| IBIS file stm32h562_563_573_ufbga201.ibs
[IBIS ver] 4.2
[File name] stm32h562_563_573_ufbga201.ibs
[File Rev] 1.1
[Date] 07-05-2024
[Source] Data Created at STMicroelectronics
[Notes]  File originated from ELDO simulations.
[Disclaimer]  This information is for modeling purpose only and is
   not guaranteed. The information is subject to change without
   notice.
[Copyright] Copyright 2024 STMicroelectronics Inc.
|   Component stm32h562_563_573_ufbga201
[Component] stm32h562_563_573_ufbga201
[Manufacturer] STMicroelectronics
[Package]
| variable   typ   min   max
R_pkg  0  NA  NA
L_pkg  0  NA  NA
C_pkg  0  NA  NA
[Pin]   signal_name   model_name
A1  PE3  io8_ft_i3c_spi
A2  PE2  io8_ft_i3c_spi
A3  PE1  io8_ft_i3c_spi
A4  PE0  io8_ft_i3c_spi
A5  PB8  io8_ft_i3c_spi
A6  PB5  io8_ft_i3c_spi
A7  PG14  io8_ft_i3c_spi
A8  PG13  io8_ft_i3c_spi
A9  PB4  io8_ft_i3c_spi
A10  PB3  io8_ft_i3c_spi
A11  PD7  io8_ft_i3c_spi
A12  PC12  io8_ft_i3c_spi
A13  PA15  io8_ft_i3c_spi
A14  PA14  io8_ft_i3c_spi
A15  PA13  io8_ft_i3c_spi
B1  PE4  io8_ft_i3c_spi
B2  PE5  io8_ft_i3c_spi
B3  PE6  io8_ft_i3c_spi
B4  PB9  io8_ft_i3c_spi
B5  PB7  io8_ft_i3c_spi
B6  PB6  io8_ft_i3c_spi
B7  PG15  io8_ft_i3c_spi
B8  PG12  io8_ft_i3c_spi
B9  PG11  io8_ft_i3c_spi
B10  PG10  io8_ft_i3c_spi
B11  PD6  io8_ft_i3c_spi
B12  PD0  io8_ft_i3c_spi
B13  PC11  io8_ft_i3c_spi
B14  PC10  io8_ft_i3c_spi
B15  PA12  io8usb_ft_i3c_spi_phy
C1  VBAT  power
C2  PI7  io8_ft_i3c_spi
C3  PI6  io8_ft_i3c_spi
C4  PI5  io8_ft_i3c_spi
C5  VDD  power
C6  VCAP  nc
C7  VDD  power
C8  VDDIO2  power
C9  VDD  power
C10  PG9  io8_ft_i3c_spi
C11  PD5  io8_ft_i3c_spi
C12  PD1  io8_ft_i3c_spi
C13  PI3  io8_ft_i3c_spi
C14  PI2  io8_ft_i3c_spi
C15  PA11  io8usb_ft_i3c_spi_phy
D1  PC13  io8_ft_i3c_spi
D2  PI8  io8_ft_i3c_spi
D3  PI9  io8_ft_i3c_spi
D4  PI4  io8_ft_i3c_spi
D5  VSS  gnd
D6  BOOT0  vpphv
D7  VSS  gnd
D8  VSS  gnd
D9  VSS  gnd
D10  PD4  io8_ft_i3c_spi
D11  PD3  io8_ft_i3c_spi
D12  PD2  io8_ft_i3c_spi
D13  PH15  io8_ft_i3c_spi
D14  PI1  io8_ft_i3c_spi
D15  PA10  io8_ft_i3c_spi
E1  PC14-OSC32_IN  io8_ft_i3c_spi
E2  PF0  io8_ft_i3c_spi
E3  PI10  io8_ft_i3c_spi
E4  PI11  io8_ft_i3c_spi
E12  PH13  io8_ft_i3c_spi
E13  PH14  io8_ft_i3c_spi
E14  PI0  io8_ft_i3c_spi
E15  PA9  io8_ft_i3c_spi
F1  PC15-OSC32_OUT  io8_ft_i3c_spi
F2  VSS  gnd
F3  VDD  power
F4  PH2  io8_ft_i3c_spi
F6  VSS  gnd
F7  VSS  gnd
F8  VSS  gnd
F9  VSS  gnd
F10  VSS  gnd
F12  VSS  gnd
F13  VDD  power
F14  PC9  io8_ft_i3c_spi
F15  PA8  io8_ft_i3c_spi
G1  PH0-OSC_IN  io8_ft_i3c_spi
G2  VSS  gnd
G3  VDD  power
G4  PH3  io8_ft_i3c_spi
G6  VSS  gnd
G7  VSS  gnd
G8  VSS  gnd
G9  VSS  gnd
G10  VSS  gnd
G12  VSS  gnd
G13  VDD  power
G14  PC8  io8_ft_i3c_spi
G15  PC7  io8_ft_i3c_spi
H1  PH1-OSC_OUT  io8_ft_i3c_spi
H2  PF2  io8_ft_i3c_spi
H3  PF1  io8_ft_i3c_spi
H4  PH4  io8_ft_i3c_spi
H6  VSS  gnd
H7  VSS  gnd
H8  VSS  gnd
H9  VSS  gnd
H10  VSS  gnd
H12  VSS  gnd
H13  VDDUSB  power
H14  PG8  io8_ft_i3c_spi
H15  PC6  io8_ft_i3c_spi
J1  NRST  ioreset_ft_v33
J2  PF3  io8_ft_i3c_spi
J3  PF4  io8_ft_i3c_spi
J4  PH5  io8_ft_i3c_spi
J6  VSS  gnd
J7  VSS  gnd
J8  VSS  gnd
J9  VSS  gnd
J10  VSS  gnd
J12  VDD  power
J13  VDD  power
J14  PG7  io8_ft_i3c_spi
J15  PG6  io8_ft_i3c_spi
K1  PF7  io8_ft_i3c_spi
K2  PF6  io8_ft_i3c_spi
K3  PF5  io8_ft_i3c_spi
K4  VDD  power
K6  VSS  gnd
K7  VSS  gnd
K8  VSS  gnd
K9  VSS  gnd
K10  VSS  gnd
K12  PH12  io8_ft_i3c_spi
K13  PG5  io8_ft_i3c_spi
K14  PG4  io8_ft_i3c_spi
K15  PG3  io8_ft_i3c_spi
L1  PF10  io8_ft_i3c_spi
L2  PF9  io8_ft_i3c_spi
L3  PF8  io8_ft_i3c_spi
L4  VSS  gnd
L12  PH11  io8_ft_i3c_spi
L13  PH10  io8_ft_i3c_spi
L14  PD15  io8_ft_i3c_spi
L15  PG2  io8_ft_i3c_spi
M1  VSSA  nc
M2  PC0  io8_ft_spi
M3  PC1  io8_ft_spi
M4  PC2  io8_ft_spi
M5  PC3  io8_ft_spi
M6  PB2  io8_ft_i3c_spi
M7  PG1  io8_ft_i3c_spi
M8  VSS  gnd
M9  VSS  gnd
M10  VCAP  nc
M11  PH6  io8_ft_i3c_spi
M12  PH8  io8_ft_i3c_spi
M13  PH9  io8_ft_i3c_spi
M14  PD14  io8_ft_i3c_spi
M15  PD13  io8_ft_i3c_spi
N1  VREFM  nc
N2  PA1  io8_ft_spi_tamp
N3  PA0  io8_ft_spi
N4  PA4  io8_ft_spi
N5  PC4  io8_ft_spi
N6  PF13  io8_ft_spi
N7  PG0  io8_ft_i3c_spi
N8  VDD  power
N9  VDD  power
N10  VDD  power
N11  PE13  io8_ft_i3c_spi
N12  PH7  io8_ft_i3c_spi
N13  PD12  io8_ft_i3c_spi
N14  PD11  io8_ft_i3c_spi
N15  PD10  io8_ft_i3c_spi
P1  VREFP  nc
P2  PA2  io8_ft_spi
P3  PA6  io8_ft_spi
P4  PA5  io8_ft_spi
P5  PC5  io8_ft_spi
P6  PF12  io8_ft_spi
P7  PF15  io8_ft_i3c_spi
P8  PE8  io8_ft_i3c_spi
P9  PE9  io8_ft_i3c_spi
P10  PE11  io8_ft_i3c_spi
P11  PE14  io8_ft_i3c_spi
P12  PB12  io8_ft_i3c_spi
|P13  PB13  io8usb_ft_pd
P13  PB13  nc
P14  PD9  io8_ft_i3c_spi
P15  PD8  io8_ft_i3c_spi
R1  VDDA  nc
R2  PA3  io8_ft_spi
R3  PA7  io8_ft_spi
R4  PB1  io8_ft_spi
R5  PB0  io8_ft_spi
R6  PF11  io8_ft_spi
R7  PF14  io8_ft_spi
R8  PE7  io8_ft_i3c_spi
R9  PE10  io8_ft_i3c_spi
R10  PE12  io8_ft_i3c_spi
R11  PE15  io8_ft_i3c_spi
R12  PB10  io8_ft_i3c_spi
R13  PB11  io8_ft_i3c_spi
|R14  PB14  io8usb_ft_pd
R14  PB14  nc
R15  PB15  io8_ft_spi
[Package Model]   484-ufbga-10x10-201-ldo-221014
[Pin Mapping]   pulldown_ref   pullup_ref   | Comment
A1  gndio  vddiom
A2  gndio  vddiom
A3  gndio  vddiom  | Depending on IO usage
| A3  gndio  vddmmc  | Depending on IO usage
A4  gndio  vddiom  | Depending on IO usage
| A4  gndio  vddmmc  | Depending on IO usage
A5  gndio  vddiom  | Depending on IO usage
| A5  gndio  vddmmc  | Depending on IO usage
A6  gndio  vddiom  | Depending on IO usage
| A6  gndio  vddmmc  | Depending on IO usage
A7  gndio  vddiom  | Depending on IO usage
| A7  gndio  vddmmc  | Depending on IO usage
A8  gndio  vddiom  | Depending on IO usage
| A8  gndio  vddmmc  | Depending on IO usage
A9  gndio  vddiom  | Depending on IO usage
| A9  gndio  vddmmc  | Depending on IO usage
A10  gndio  vddiom  | Depending on IO usage
| A10  gndio  vddmmc  | Depending on IO usage
A11  gndio  vddiom  | Depending on IO usage
| A11  gndio  vddmmc  | Depending on IO usage
A12  gndio  vddiom
A13  gndio  vddiom
A14  gndio  vddiom
A15  gndio  vddiom  | Depending on IO usage
| A15  gndio  vddusb  | Depending on IO usage
B1  gndio  vddiom
B2  gndio  vddiom
B3  gndio  vddiom
B4  gndio  vddiom  | Depending on IO usage
| B4  gndio  vddmmc  | Depending on IO usage
B5  gndio  vddiom  | Depending on IO usage
| B5  gndio  vddmmc  | Depending on IO usage
B6  gndio  vddiom  | Depending on IO usage
| B6  gndio  vddmmc  | Depending on IO usage
B7  gndio  vddiom  | Depending on IO usage
| B7  gndio  vddmmc  | Depending on IO usage
B8  gndio  vddiom  | Depending on IO usage
| B8  gndio  vddmmc  | Depending on IO usage
B9  gndio  vddiom  | Depending on IO usage
| B9  gndio  vddmmc  | Depending on IO usage
B10  gndio  vddiom  | Depending on IO usage
| B10  gndio  vddmmc  | Depending on IO usage
B11  gndio  vddiom  | Depending on IO usage
| B11  gndio  vddmmc  | Depending on IO usage
B12  gndio  vddiom
B13  gndio  vddiom
B14  gndio  vddiom
B15  gndio  vddiom  | Depending on IO usage
| B15  gndio  vddusb  | Depending on IO usage
C1  nc  vsw
C2  gndio  vddiom
C3  gndio  vddiom
C4  gndio  vddiom
C5  nc  vddiom
C6  nc  nc
C7  nc  vddiom
C8  nc  vddmmc
C9  nc  vddiom
C10  gndio  vddiom  | Depending on IO usage
| C10  gndio  vddmmc  | Depending on IO usage
C11  gndio  vddiom
C12  gndio  vddiom
C13  gndio  vddiom
C14  gndio  vddiom
C15  gndio  vddiom  | Depending on IO usage
| C15  gndio  vddusb  | Depending on IO usage
D1  gndio  vddiom  | Depending on IO usage
| D1  gndio  vsw  | Depending on IO usage
D2  gndio  vddiom  | Depending on IO usage
| D2  gndio  vsw  | Depending on IO usage
D3  gndio  vddiom
D4  gndio  vddiom
D5  gndio  nc
D6  gndio  vddiom  | Depending on IO usage
| D6  gndio  vddmmc  | Depending on IO usage
D7  gndio  nc
D8  gndio  nc
D9  gndio  nc
D10  gndio  vddiom
D11  gndio  vddiom
D12  gndio  vddiom
D13  gndio  vddiom
D14  gndio  vddiom
D15  gndio  vddiom  | Depending on IO usage
| D15  gndio  vddusb  | Depending on IO usage
E1  gndio  vddiom  | Depending on IO usage
| E1  gndio  vsw  | Depending on IO usage
E2  gndio  vddiom
E3  gndio  vddiom
E4  gndio  vddiom
E12  gndio  vddiom
E13  gndio  vddiom
E14  gndio  vddiom
E15  gndio  vddiom  | Depending on IO usage
| E15  gndio  vddusb  | Depending on IO usage
F1  gndio  vddiom  | Depending on IO usage
| F1  gndio  vsw  | Depending on IO usage
F2  gndio  nc
F3  nc  vddiom
F4  gndio  vddiom
F6  gndio  nc
F7  gndio  nc
F8  gndio  nc
F9  gndio  nc
F10  gndio  nc
F12  gndio  nc
F13  nc  vddiom
F14  gndio  vddiom
F15  gndio  vddiom
G1  gndio  vddiom
G2  gndio  nc
G3  nc  vddiom
G4  gndio  vddiom
G6  gndio  nc
G7  gndio  nc
G8  gndio  nc
G9  gndio  nc
G10  gndio  nc
G12  gndio  nc
G13  nc  vddiom
G14  gndio  vddiom
G15  gndio  vddiom
H1  gndio  vddiom
H2  gndio  vddiom
H3  gndio  vddiom
H4  gndio  vddiom
H6  gndio  nc
H7  gndio  nc
H8  gndio  nc
H9  gndio  nc
H10  gndio  nc
H12  gndio  nc
H13  nc  vddusb
H14  gndio  vddiom
H15  gndio  vddiom
J1  gndio  vddiom
J2  gndio  vddiom
J3  gndio  vddiom
J4  gndio  vddiom
J6  gndio  nc
J7  gndio  nc
J8  gndio  nc
J9  gndio  nc
J10  gndio  nc
J12  nc  vddiom
J13  nc  vddiom
J14  gndio  vddiom
J15  gndio  vddiom
K1  gndio  vddiom
K2  gndio  vddiom
K3  gndio  vddiom
K4  nc  vddiom
K6  gndio  nc
K7  gndio  nc
K8  gndio  nc
K9  gndio  nc
K10  gndio  nc
K12  gndio  vddiom
K13  gndio  vddiom
K14  gndio  vddiom
K15  gndio  vddiom
L1  gndio  vddiom
L2  gndio  vddiom
L3  gndio  vddiom
L4  gndio  nc
L12  gndio  vddiom
L13  gndio  vddiom
L14  gndio  vddiom
L15  gndio  vddiom
M1  nc  nc
M2  gndio  vddiom
M3  gndio  vddiom
M4  gndio  vddiom
M5  gndio  vddiom
M6  gndio  vddiom
M7  gndio  vddiom
M8  gndio  nc
M9  gndio  nc
M10  nc  nc
M11  gndio  vddiom
M12  gndio  vddiom
M13  gndio  vddiom
M14  gndio  vddiom
M15  gndio  vddiom
N1  nc  nc
N2  gndio  vddiom
N3  gndio  vddiom
N4  gndio  vddiom
N5  gndio  vddiom
N6  gndio  vddiom
N7  gndio  vddiom
N8  nc  vddiom
N9  nc  vddiom
N10  nc  vddiom
N11  gndio  vddiom
N12  gndio  vddiom
N13  gndio  vddiom
N14  gndio  vddiom
N15  gndio  vddiom
P1  nc  nc
P2  gndio  vddiom
P3  gndio  vddiom
P4  gndio  vddiom
P5  gndio  vddiom
P6  gndio  vddiom
P7  gndio  vddiom
P8  gndio  vddiom
P9  gndio  vddiom
P10  gndio  vddiom
P11  gndio  vddiom
P12  gndio  vddiom
P13  nc nc
|P13  gndio  vddiom
P14  gndio  vddiom
P15  gndio  vddiom
R1  nc  nc
R2  gndio  vddiom
R3  gndio  vddiom
R4  gndio  vddiom
R5  gndio  vddiom
R6  gndio  vddiom
R7  gndio  vddiom
R8  gndio  vddiom
R9  gndio  vddiom
R10  gndio  vddiom
R11  gndio  vddiom
R12  gndio  vddiom
R13  gndio  vddiom
|R14  gndio  vddiom
R14  nc nc
R15  gndio  vddiom
[Model Selector] io8_ft_i3c_spi
io8_ft_spi_ls_1v2 "io8_ft spi low speed @ 1.2V"
io8_ft_spi_ls_1v8 "io8_ft spi low speed @ 1.8V"
io8_ft_spi_ls_3v3 "io8_ft spi low speed @ 3.3V"
io8_ft_spi_ms_1v2 "io8_ft spi med speed @ 1.2V"
io8_ft_spi_ms_1v8 "io8_ft spi med speed @ 1.8V"
io8_ft_spi_ms_3v3 "io8_ft spi med speed @ 3.3V"
io8_ft_spi_fs_1v2 "io8_ft spi fast speed @ 1.2V"
io8_ft_spi_fs_1v8 "io8_ft spi fast speed @ 1.8V"
io8_ft_spi_fs_3v3 "io8_ft spi fast speed @ 3.3V"
io8_ft_spi_hs_1v2 "io8_ft spi high speed @ 1.2V"
io8_ft_spi_hs_1v8 "io8_ft spi high speed @ 1.8V"
io8_ft_spi_hs_3v3 "io8_ft spi high speed @ 3.3V"
io8_ft_hslv_spi_ls_1v2 "io8_ft spi hslv low speed @ 1.2V"
io8_ft_hslv_spi_ls_1v8 "io8_ft spi hslv low speed @ 1.8V"
io8_ft_hslv_spi_ls_2v5 "io8_ft spi hslv low speed @ 2.5V"
io8_ft_hslv_spi_ms_1v2 "io8_ft spi hslv med speed @ 1.2V"
io8_ft_hslv_spi_ms_1v8 "io8_ft spi hslv med speed @ 1.8V"
io8_ft_hslv_spi_ms_2v5 "io8_ft spi hslv med speed @ 2.5V"
io8_ft_hslv_spi_fs_1v2 "io8_ft spi hslv fast speed @ 1.2V"
io8_ft_hslv_spi_fs_1v8 "io8_ft spi hslv fast speed @ 1.8V"
io8_ft_hslv_spi_fs_2v5 "io8_ft spi hslv fast speed @ 2.5V"
io8_ft_hslv_spi_hs_1v2 "io8_ft spi hslv high speed @ 1.2V"
io8_ft_hslv_spi_hs_1v8 "io8_ft spi hslv high speed @ 1.8V"
io8_ft_hslv_spi_hs_2v5 "io8_ft spi hslv high speed @ 2.5V"
io8_ft_i3c_spi_ls_1v2 "io8_ft i3c spi open-drain low speed @ 1.2V"
io8_ft_i3c_spi_ls_1v8 "io8_ft i3c spi open-drain low speed @ 1.8V"
io8_ft_i3c_spi_ls_3v3 "io8_ft i3c spi open-drain low speed @ 3.3V"
io8_ft_i3c_spi_ms_1v2 "io8_ft i3c spi open-drain med speed @ 1.2V"
io8_ft_i3c_spi_ms_1v8 "io8_ft i3c spi open-drain med speed @ 1.8V"
io8_ft_i3c_spi_ms_3v3 "io8_ft i3c spi open-drain med speed @ 3.3V"
io8_ft_i3c_spi_fs_1v2 "io8_ft i3c spi open-drain fast speed @ 1.2V"
io8_ft_i3c_spi_fs_1v8 "io8_ft i3c spi open-drain fast speed @ 1.8V"
io8_ft_i3c_spi_fs_3v3 "io8_ft i3c spi open-drain fast speed @ 3.3V"
io8_ft_i3c_spi_hs_1v2 "io8_ft i3c spi open-drain high speed @ 1.2V"
io8_ft_i3c_spi_hs_1v8 "io8_ft i3c spi open-drain high speed @ 1.8V"
io8_ft_i3c_spi_hs_3v3 "io8_ft i3c spi open-drain high speed @ 3.3V"
io8_ft_hslv_i3c_spi_ls_1v2 "io8_ft hslv i3c spi open-drain low speed @ 1.2V"
io8_ft_hslv_i3c_spi_ls_1v8 "io8_ft hslv i3c spi open-drain low speed @ 1.8V"
io8_ft_hslv_i3c_spi_ls_2v5 "io8_ft hslv i3c spi open-drain low speed @ 2.5V"
io8_ft_hslv_i3c_spi_ms_1v2 "io8_ft hslv i3c spi open-drain med speed @ 1.2V"
io8_ft_hslv_i3c_spi_ms_1v8 "io8_ft hslv i3c spi open-drain med speed @ 1.8V"
io8_ft_hslv_i3c_spi_ms_2v5 "io8_ft hslv i3c spi open-drain med speed @ 2.5V"
io8_ft_hslv_i3c_spi_fs_1v2 "io8_ft hslv i3c spi open-drain fast speed @ 1.2V"
io8_ft_hslv_i3c_spi_fs_1v8 "io8_ft hslv i3c spi open-drain fast speed @ 1.8V"
io8_ft_hslv_i3c_spi_fs_2v5 "io8_ft hslv i3c spi open-drain fast speed @ 2.5V"
io8_ft_hslv_i3c_spi_hs_1v2 "io8_ft hslv i3c spi open-drain high speed @ 1.2V"
io8_ft_hslv_i3c_spi_hs_1v8 "io8_ft hslv i3c spi open-drain high speed @ 1.8V"
io8_ft_hslv_i3c_spi_hs_2v5 "io8_ft hslv i3c spi open-drain high speed @ 2.5V"
io8_ft_i3c_fmp_spi_3v3 "io8_ft i3c fm+ spi open-drain @ 3.3V"
io8_ft_i3c_fmp_spi_1v8 "io8_ft i3c fm+ spi open-drain @ 1.8V"
io8_ft_i3c_fmp_spi_1v2 "io8_ft i3c fm+ spi open-drain @ 1.2V"
[Model Selector] io8_ft_spi
io8_ft_spi_ls_1v2 "io8_ft spi low speed @ 1.2V"
io8_ft_spi_ls_1v8 "io8_ft spi low speed @ 1.8V"
io8_ft_spi_ls_3v3 "io8_ft spi low speed @ 3.3V"
io8_ft_spi_ms_1v2 "io8_ft spi med speed @ 1.2V"
io8_ft_spi_ms_1v8 "io8_ft spi med speed @ 1.8V"
io8_ft_spi_ms_3v3 "io8_ft spi med speed @ 3.3V"
io8_ft_spi_fs_1v2 "io8_ft spi fast speed @ 1.2V"
io8_ft_spi_fs_1v8 "io8_ft spi fast speed @ 1.8V"
io8_ft_spi_fs_3v3 "io8_ft spi fast speed @ 3.3V"
io8_ft_spi_hs_1v2 "io8_ft spi high speed @ 1.2V"
io8_ft_spi_hs_1v8 "io8_ft spi high speed @ 1.8V"
io8_ft_spi_hs_3v3 "io8_ft spi high speed @ 3.3V"
io8_ft_hslv_spi_ls_1v2 "io8_ft spi hslv low speed @ 1.2V"
io8_ft_hslv_spi_ls_1v8 "io8_ft spi hslv low speed @ 1.8V"
io8_ft_hslv_spi_ls_2v5 "io8_ft spi hslv low speed @ 2.5V"
io8_ft_hslv_spi_ms_1v2 "io8_ft spi hslv med speed @ 1.2V"
io8_ft_hslv_spi_ms_1v8 "io8_ft spi hslv med speed @ 1.8V"
io8_ft_hslv_spi_ms_2v5 "io8_ft spi hslv med speed @ 2.5V"
io8_ft_hslv_spi_fs_1v2 "io8_ft spi hslv fast speed @ 1.2V"
io8_ft_hslv_spi_fs_1v8 "io8_ft spi hslv fast speed @ 1.8V"
io8_ft_hslv_spi_fs_2v5 "io8_ft spi hslv fast speed @ 2.5V"
io8_ft_hslv_spi_hs_1v2 "io8_ft spi hslv high speed @ 1.2V"
io8_ft_hslv_spi_hs_1v8 "io8_ft spi hslv high speed @ 1.8V"
io8_ft_hslv_spi_hs_2v5 "io8_ft spi hslv high speed @ 2.5V"
[Model Selector] io8_ft_spi_tamp
io8_ft_spi_ls_1v2 "io8_ft spi low speed @ 1.2V"
io8_ft_spi_ls_1v8 "io8_ft spi low speed @ 1.8V"
io8_ft_spi_ls_3v3 "io8_ft spi low speed @ 3.3V"
io8_ft_spi_ms_1v2 "io8_ft spi med speed @ 1.2V"
io8_ft_spi_ms_1v8 "io8_ft spi med speed @ 1.8V"
io8_ft_spi_ms_3v3 "io8_ft spi med speed @ 3.3V"
io8_ft_spi_fs_1v2 "io8_ft spi fast speed @ 1.2V"
io8_ft_spi_fs_1v8 "io8_ft spi fast speed @ 1.8V"
io8_ft_spi_fs_3v3 "io8_ft spi fast speed @ 3.3V"
io8_ft_spi_hs_1v2 "io8_ft spi high speed @ 1.2V"
io8_ft_spi_hs_1v8 "io8_ft spi high speed @ 1.8V"
io8_ft_spi_hs_3v3 "io8_ft spi high speed @ 3.3V"
io8_ft_hslv_spi_ls_1v2 "io8_ft spi hslv low speed @ 1.2V"
io8_ft_hslv_spi_ls_1v8 "io8_ft spi hslv low speed @ 1.8V"
io8_ft_hslv_spi_ls_2v5 "io8_ft spi hslv low speed @ 2.5V"
io8_ft_hslv_spi_ms_1v2 "io8_ft spi hslv med speed @ 1.2V"
io8_ft_hslv_spi_ms_1v8 "io8_ft spi hslv med speed @ 1.8V"
io8_ft_hslv_spi_ms_2v5 "io8_ft spi hslv med speed @ 2.5V"
io8_ft_hslv_spi_fs_1v2 "io8_ft spi hslv fast speed @ 1.2V"
io8_ft_hslv_spi_fs_1v8 "io8_ft spi hslv fast speed @ 1.8V"
io8_ft_hslv_spi_fs_2v5 "io8_ft spi hslv fast speed @ 2.5V"
io8_ft_hslv_spi_hs_1v2 "io8_ft spi hslv high speed @ 1.2V"
io8_ft_hslv_spi_hs_1v8 "io8_ft spi hslv high speed @ 1.8V"
io8_ft_hslv_spi_hs_2v5 "io8_ft spi hslv high speed @ 2.5V"
io8_ft_tamp_v33_1v2 "io8_ft tamp V33 @ 1.2V"
io8_ft_tamp_v33_1v8 "io8_ft tamp V33 @ 1.2V"
io8_ft_tamp_v33_3v3 "io8_ft tamp V33 @ 1.2V"
[Model Selector] io8usb_ft_i3c_spi_phy
io8_ft_spi_ls_1v2 "io8_ft spi low speed @ 1.2V"
io8_ft_spi_ls_1v8 "io8_ft spi low speed @ 1.8V"
io8_ft_spi_ls_3v3 "io8_ft spi low speed @ 3.3V"
io8_ft_spi_ms_1v2 "io8_ft spi med speed @ 1.2V"
io8_ft_spi_ms_1v8 "io8_ft spi med speed @ 1.8V"
io8_ft_spi_ms_3v3 "io8_ft spi med speed @ 3.3V"
io8_ft_spi_fs_1v2 "io8_ft spi fast speed @ 1.2V"
io8_ft_spi_fs_1v8 "io8_ft spi fast speed @ 1.8V"
io8_ft_spi_fs_3v3 "io8_ft spi fast speed @ 3.3V"
io8_ft_spi_hs_1v2 "io8_ft spi high speed @ 1.2V"
io8_ft_spi_hs_1v8 "io8_ft spi high speed @ 1.8V"
io8_ft_spi_hs_3v3 "io8_ft spi high speed @ 3.3V"
io8_ft_hslv_spi_ls_1v2 "io8_ft spi hslv low speed @ 1.2V"
io8_ft_hslv_spi_ls_1v8 "io8_ft spi hslv low speed @ 1.8V"
io8_ft_hslv_spi_ls_2v5 "io8_ft spi hslv low speed @ 2.5V"
io8_ft_hslv_spi_ms_1v2 "io8_ft spi hslv med speed @ 1.2V"
io8_ft_hslv_spi_ms_1v8 "io8_ft spi hslv med speed @ 1.8V"
io8_ft_hslv_spi_ms_2v5 "io8_ft spi hslv med speed @ 2.5V"
io8_ft_hslv_spi_fs_1v2 "io8_ft spi hslv fast speed @ 1.2V"
io8_ft_hslv_spi_fs_1v8 "io8_ft spi hslv fast speed @ 1.8V"
io8_ft_hslv_spi_fs_2v5 "io8_ft spi hslv fast speed @ 2.5V"
io8_ft_hslv_spi_hs_1v2 "io8_ft spi hslv high speed @ 1.2V"
io8_ft_hslv_spi_hs_1v8 "io8_ft spi hslv high speed @ 1.8V"
io8_ft_hslv_spi_hs_2v5 "io8_ft spi hslv high speed @ 2.5V"
io8_ft_i3c_spi_ls_1v2 "io8_ft i3c spi open-drain low speed @ 1.2V"
io8_ft_i3c_spi_ls_1v8 "io8_ft i3c spi open-drain low speed @ 1.8V"
io8_ft_i3c_spi_ls_3v3 "io8_ft i3c spi open-drain low speed @ 3.3V"
io8_ft_i3c_spi_ms_1v2 "io8_ft i3c spi open-drain med speed @ 1.2V"
io8_ft_i3c_spi_ms_1v8 "io8_ft i3c spi open-drain med speed @ 1.8V"
io8_ft_i3c_spi_ms_3v3 "io8_ft i3c spi open-drain med speed @ 3.3V"
io8_ft_i3c_spi_fs_1v2 "io8_ft i3c spi open-drain fast speed @ 1.2V"
io8_ft_i3c_spi_fs_1v8 "io8_ft i3c spi open-drain fast speed @ 1.8V"
io8_ft_i3c_spi_fs_3v3 "io8_ft i3c spi open-drain fast speed @ 3.3V"
io8_ft_i3c_spi_hs_1v2 "io8_ft i3c spi open-drain high speed @ 1.2V"
io8_ft_i3c_spi_hs_1v8 "io8_ft i3c spi open-drain high speed @ 1.8V"
io8_ft_i3c_spi_hs_3v3 "io8_ft i3c spi open-drain high speed @ 3.3V"
io8_ft_hslv_i3c_spi_ls_1v2 "io8_ft hslv i3c spi open-drain low speed @ 1.2V"
io8_ft_hslv_i3c_spi_ls_1v8 "io8_ft hslv i3c spi open-drain low speed @ 1.8V"
io8_ft_hslv_i3c_spi_ls_2v5 "io8_ft hslv i3c spi open-drain low speed @ 2.5V"
io8_ft_hslv_i3c_spi_ms_1v2 "io8_ft hslv i3c spi open-drain med speed @ 1.2V"
io8_ft_hslv_i3c_spi_ms_1v8 "io8_ft hslv i3c spi open-drain med speed @ 1.8V"
io8_ft_hslv_i3c_spi_ms_2v5 "io8_ft hslv i3c spi open-drain med speed @ 2.5V"
io8_ft_hslv_i3c_spi_fs_1v2 "io8_ft hslv i3c spi open-drain fast speed @ 1.2V"
io8_ft_hslv_i3c_spi_fs_1v8 "io8_ft hslv i3c spi open-drain fast speed @ 1.8V"
io8_ft_hslv_i3c_spi_fs_2v5 "io8_ft hslv i3c spi open-drain fast speed @ 2.5V"
io8_ft_hslv_i3c_spi_hs_1v2 "io8_ft hslv i3c spi open-drain high speed @ 1.2V"
io8_ft_hslv_i3c_spi_hs_1v8 "io8_ft hslv i3c spi open-drain high speed @ 1.8V"
io8_ft_hslv_i3c_spi_hs_2v5 "io8_ft hslv i3c spi open-drain high speed @ 2.5V"
io8_ft_i3c_fmp_spi_3v3 "io8_ft i3c fm+ spi open-drain @ 3.3V"
io8_ft_i3c_fmp_spi_1v8 "io8_ft i3c fm+ spi open-drain @ 1.8V"
io8_ft_i3c_fmp_spi_1v2 "io8_ft i3c fm+ spi open-drain @ 1.2V"
io8usb_ft_phy_ls_2v5 "iousb ft low speed @ 2.5V"
io8usb_ft_phy_ls_3v3 "iousb ft low speed @ 3.3V"
io8usb_ft_phy_fs_2v5 "iousb ft fast speed @ 2.5V"
io8usb_ft_phy_fs_3v3 "iousb ft fast speed @ 3.3V"
[Model Selector] ioreset_ft_v33
ioreset_ft_v33_1v2 "Reset PAD. 5V tolerant. 1.2V range"
ioreset_ft_v33_1v8 "Reset PAD. 5V tolerant. 1.8V range"
ioreset_ft_v33_3v3 "Reset PAD. 5V tolerant. 3.3V range"
[Model Selector] vpphv
vpphv_1v2 "Flash Test cell v33 = 1.2 V range"
vpphv_1v8 "Flash Test cell v33 = 1.8 V range"
vpphv_3v3 "Flash Test cell v33 = 3.3 V range"
[Define Package Model]  484-ufbga-10x10-201-ldo-221014
[Manufacturer]  unknown
[OEM]  unknown
[Description]  unknown
[Number Of Pins]  153
[Pin Numbers]
| Pin Name Terminal   Net Name   Starting Node   Ending Node
D6 | BOOT0
J1 | NRST
N3 | PA0
N2 | PA1
P2 | PA2
R2 | PA3
N4 | PA4
P4 | PA5
P3 | PA6
R3 | PA7
F15 | PA8
E15 | PA9
D15 | PA10
C15 | PA11
B15 | PA12
A15 | PA13
A14 | PA14
A13 | PA15
R5 | PB0
R4 | PB1
M6 | PB2
A10 | PB3
A9 | PB4
A6 | PB5
B6 | PB6
B5 | PB7
A5 | PB8
B4 | PB9
R12 | PB10
R13 | PB11
P12 | PB12
P13 | PB13
R14 | PB14
R15 | PB15
M2 | PC0
M3 | PC1
M4 | PC2
M5 | PC3
N5 | PC4
P5 | PC5
H15 | PC6
G15 | PC7
G14 | PC8
F14 | PC9
B14 | PC10
B13 | PC11
A12 | PC12
D1 | PC13
E1 | PC14-OSC32_IN
F1 | PC15-OSC32_OUT
B12 | PD0
C12 | PD1
D12 | PD2
D11 | PD3
D10 | PD4
C11 | PD5
B11 | PD6
A11 | PD7
P15 | PD8
P14 | PD9
N15 | PD10
N14 | PD11
N13 | PD12
M15 | PD13
M14 | PD14
L14 | PD15
A4 | PE0
A3 | PE1
A2 | PE2
A1 | PE3
B1 | PE4
B2 | PE5
B3 | PE6
R8 | PE7
P8 | PE8
P9 | PE9
R9 | PE10
P10 | PE11
R10 | PE12
N11 | PE13
P11 | PE14
R11 | PE15
E2 | PF0
H3 | PF1
H2 | PF2
J2 | PF3
J3 | PF4
K3 | PF5
K2 | PF6
K1 | PF7
L3 | PF8
L2 | PF9
L1 | PF10
R6 | PF11
P6 | PF12
N6 | PF13
R7 | PF14
P7 | PF15
N7 | PG0
M7 | PG1
L15 | PG2
K15 | PG3
K14 | PG4
K13 | PG5
J15 | PG6
J14 | PG7
H14 | PG8
C10 | PG9
B10 | PG10
B9 | PG11
B8 | PG12
A8 | PG13
A7 | PG14
B7 | PG15
G1 | PH0-OSC_IN
H1 | PH1-OSC_OUT
F4 | PH2
G4 | PH3
H4 | PH4
J4 | PH5
M11 | PH6
N12 | PH7
M12 | PH8
M13 | PH9
L13 | PH10
L12 | PH11
K12 | PH12
E12 | PH13
E13 | PH14
D13 | PH15
E14 | PI0
D14 | PI1
C14 | PI2
C13 | PI3
D4 | PI4
C4 | PI5
C3 | PI6
C2 | PI7
D2 | PI8
D3 | PI9
E3 | PI10
E4 | PI11
C1 | VBAT
M10 | VCAP
C6 | VCAP
H13 | VDDUSB
C5 | VDD
R1 | VDDA
C8 | VDDIO2
N1 | VREFM
P1 | VREFP
D5 | VSS
M1 | VSSA
|[Merged Pins]  C5
|C7  |  VDD
|C9  |  VDD
|F3  |  VDD
|F13  |  VDD
|G3  |  VDD
|G13  |  VDD
|J12  |  VDD
|J13  |  VDD
|K4  |  VDD
|N8  |  VDD
|N9  |  VDD
|N10  |  VDD
|[Merged Pins]  D5
|D7  |  VSS
|D8  |  VSS
|D9  |  VSS
|F2  |  VSS
|F6  |  VSS
|F7  |  VSS
|F8  |  VSS
|F9  |  VSS
|F10  |  VSS
|F12  |  VSS
|G2  |  VSS
|G6  |  VSS
|G7  |  VSS
|G8  |  VSS
|G9  |  VSS
|G10  |  VSS
|G12  |  VSS
|H6  |  VSS
|H7  |  VSS
|H8  |  VSS
|H9  |  VSS
|H10  |  VSS
|H12  |  VSS
|J6  |  VSS
|J7  |  VSS
|J8  |  VSS
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[Model Data]
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[End Model Data]
[End Package Model]
|End [Component]
| Models and submodels in the file (64): io8_ft_hslv_i3c_spi_fs_1v2 (I/O_open_drain), io8_ft_hslv_i3c_spi_fs_1v8 (I/O_open_drain), io8_ft_hslv_i3c_spi_fs_2v5 (I/O_open_drain), io8_ft_hslv_i3c_spi_hs_1v2 (I/O_open_drain), io8_ft_hslv_i3c_spi_hs_1v8 (I/O_open_drain), io8_ft_hslv_i3c_spi_hs_2v5 (I/O_open_drain), io8_ft_hslv_i3c_spi_ls_1v2 (I/O_open_drain), io8_ft_hslv_i3c_spi_ls_1v8 (I/O_open_drain), io8_ft_hslv_i3c_spi_ls_2v5 (I/O_open_drain), io8_ft_hslv_i3c_spi_ms_1v2 (I/O_open_drain), io8_ft_hslv_i3c_spi_ms_1v8 (I/O_open_drain), io8_ft_hslv_i3c_spi_ms_2v5 (I/O_open_drain), io8_ft_hslv_spi_fs_1v2 (I/O), io8_ft_hslv_spi_fs_1v8 (I/O), io8_ft_hslv_spi_fs_2v5 (I/O), io8_ft_hslv_spi_hs_1v2 (I/O), io8_ft_hslv_spi_hs_1v8 (I/O), io8_ft_hslv_spi_hs_2v5 (I/O), io8_ft_hslv_spi_ls_1v2 (I/O), io8_ft_hslv_spi_ls_1v8 (I/O), io8_ft_hslv_spi_ls_2v5 (I/O), io8_ft_hslv_spi_ms_1v2 (I/O), io8_ft_hslv_spi_ms_1v8 (I/O), io8_ft_hslv_spi_ms_2v5 (I/O), io8_ft_i3c_fmp_spi_1v2 (I/O_open_drain), io8_ft_i3c_fmp_spi_1v8 (I/O_open_drain), io8_ft_i3c_fmp_spi_3v3 (I/O_open_drain), io8_ft_i3c_spi_fs_1v2 (I/O_open_drain), io8_ft_i3c_spi_fs_1v8 (I/O_open_drain), io8_ft_i3c_spi_fs_3v3 (I/O_open_drain), io8_ft_i3c_spi_hs_1v2 (I/O_open_drain), io8_ft_i3c_spi_hs_1v8 (I/O_open_drain), io8_ft_i3c_spi_hs_3v3 (I/O_open_drain), io8_ft_i3c_spi_ls_1v2 (I/O_open_drain), io8_ft_i3c_spi_ls_1v8 (I/O_open_drain), io8_ft_i3c_spi_ls_3v3 (I/O_open_drain), io8_ft_i3c_spi_ms_1v2 (I/O_open_drain), io8_ft_i3c_spi_ms_1v8 (I/O_open_drain), io8_ft_i3c_spi_ms_3v3 (I/O_open_drain), io8_ft_spi_fs_1v2 (I/O), io8_ft_spi_fs_1v8 (I/O), io8_ft_spi_fs_3v3 (I/O), io8_ft_spi_hs_1v2 (I/O), io8_ft_spi_hs_1v8 (I/O), io8_ft_spi_hs_3v3 (I/O), io8_ft_spi_ls_1v2 (I/O), io8_ft_spi_ls_1v8 (I/O), io8_ft_spi_ls_3v3 (I/O), io8_ft_spi_ms_1v2 (I/O), io8_ft_spi_ms_1v8 (I/O), io8_ft_spi_ms_3v3 (I/O), io8_ft_tamp_v33_1v2 (I/O), io8_ft_tamp_v33_1v8 (I/O), io8_ft_tamp_v33_3v3 (I/O), io8usb_ft_phy_fs_2v5 (I/O), io8usb_ft_phy_fs_3v3 (I/O), io8usb_ft_phy_ls_2v5 (I/O), io8usb_ft_phy_ls_3v3 (I/O), ioreset_ft_v33_1v2 (I/O_open_drain), ioreset_ft_v33_1v8 (I/O_open_drain), ioreset_ft_v33_3v3 (I/O_open_drain), vpphv_1v2 (Input), vpphv_1v8 (Input), vpphv_3v3 (Input)
